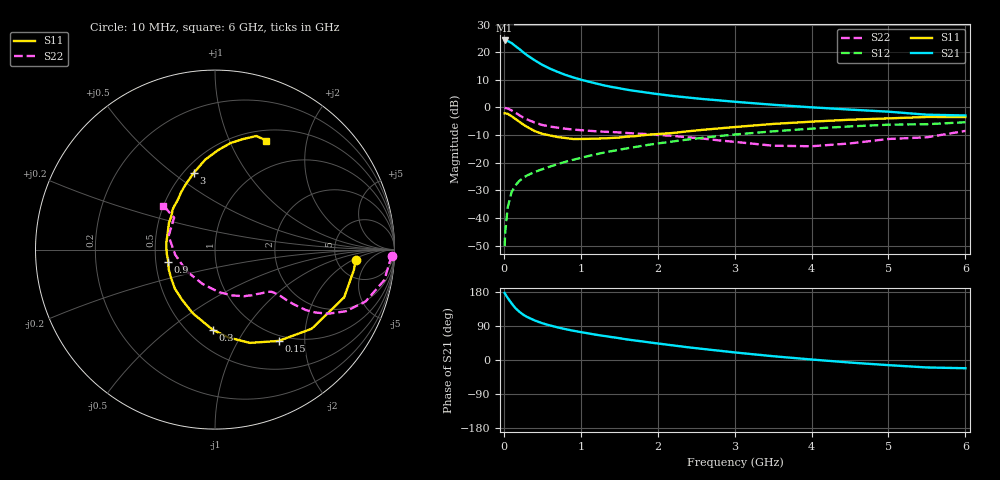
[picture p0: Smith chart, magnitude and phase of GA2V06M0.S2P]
! Infineon Technologies  Discrete & RF Semiconductors
! BF775
! Si NPN RF Bipolar Junction Transistor in SOT23
! VCE = 2 V  IC = 6 mA
! Common Emitter S-Parameters:  May  1996
# GHz  S  MA  R  50
!  f  S11  S21  S12  S22
! GHz  MAG  ANG  MAG  ANG  MAG  ANG  MAG  ANG
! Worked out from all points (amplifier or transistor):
!   36 points, 10 MHz to 6 GHz, reference 50 ohm
!   highest |S21| = 24.2 dB at 10 MHz (marker M1)
!   |S21| within 3 dB of that: start of sweep to 197.2 MHz
!   unconditionally stable (mu >= 1): 702.7 MHz to 3.917 GHz; 5.453 GHz to 5.584 GHz
!   at 250 MHz: K = 0.55, MSG = 22.8 dB, |S12| = -25.5 dB
!   at 1.4 GHz: K = 1.14, MAG = 9.3 dB, |S12| = -15.8 dB
!   at 6 GHz: K = 0.99, MSG = 1.2 dB, |S12| = -5.3 dB
!   S11 on the Smith chart (normalised r, x): 10 MHz: 7.63, -2.30; 150 MHz: 0.91, -1.51; 300 MHz: 0.65, -0.73; 900 MHz: 0.58, -0.08; 3 GHz: 0.56, +0.59; 6 GHz: 0.62, +1.38
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0.01  0.7858 -4.2  16.31 176.9  0.0031 83.2  0.9884 -2.0
0.02  0.7821 -8.4  16.11 173.3  0.0059 87.6  0.9757 -4.1
0.05  0.7672 -20.3  15.94 163.9  0.0155 79.5  0.9587 -10.2
0.1  0.6963 -39.3  14.65 149.6  0.0293 70.9  0.8875 -19.0
0.15  0.6203 -55.1  12.92 137.0  0.0388 64.6  0.8064 -25.2
0.2  0.555 -69.5  11.47 127.6  0.0468 60.6  0.727 -29.4
0.25  0.4953 -81.3  10.03 119.8  0.0531 58.0  0.6596 -32.1
0.3  0.4471 -91.6  8.852 113.8  0.0588 56.6  0.6094 -33.6
0.4  0.375 -109.5  7.157 104.5  0.0682 55.8  0.5349 -34.8
0.5  0.3332 -123.8  5.903 97.0  0.0764 56.2  0.4825 -35.2
0.6  0.312 -135.8  5.034 91.2  0.0854 56.5  0.452 -35.3
0.7  0.2916 -146.9  4.403 86.0  0.0946 57.1  0.4311 -35.6
0.9  0.2688 -165.7  3.502 77.3  0.1132 57.7  0.3991 -36.4
1.1  0.2711 177.7  2.936 70.2  0.1325 57.9  0.3797 -38.3
1.3  0.2755 165.9  2.516 63.6  0.1528 57.2  0.3648 -40.7
1.6  0.2971 149.7  2.097 54.3  0.1823 55.7  0.3457 -45.4
2.2  0.3458 126.9  1.613 38.5  0.2432 50.8  0.3061 -58.1
3  0.4423 105.7  1.27 20.0  0.3243 41.8  0.239 -84.3
3.5  0.5041 96.2  1.12 10.0  0.3703 35.5  0.2034 -110.0
4.5  0.6006 81.6  0.916 -6.7  0.4546 22.2  0.2239 -173.0
5.5  0.6736 70.0  0.74 -19.7  0.4987 7.6  0.289 142.0
6  0.6717 64.8  0.717 -21.7  0.5408 3.6  0.3771 139.6
